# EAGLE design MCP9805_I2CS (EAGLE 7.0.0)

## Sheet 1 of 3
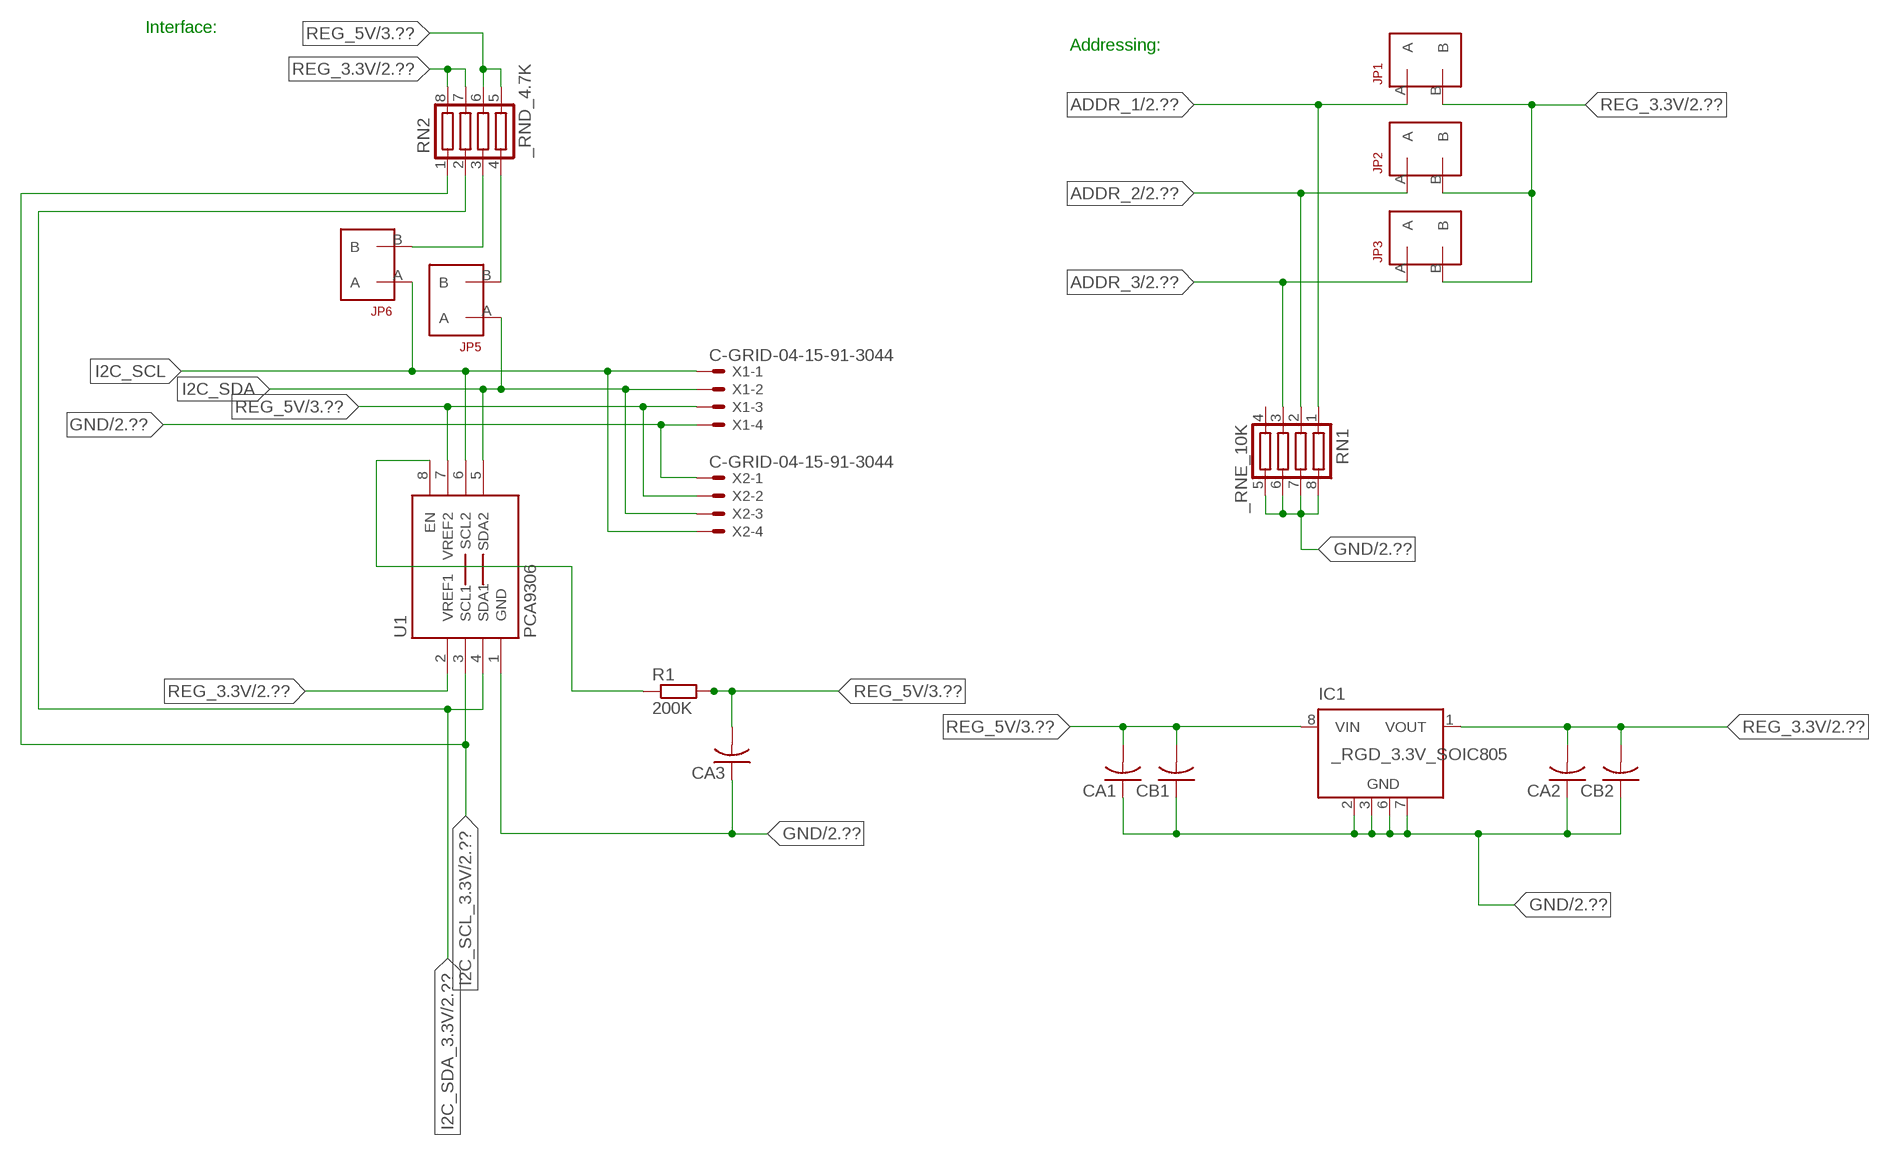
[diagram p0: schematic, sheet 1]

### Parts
CA1  CC1206KRX7R9BB104  [.1UF]
CA2  CC1206KRX7R9BB104  [.1UF]
CA3  CC1206KRX7R9BB104  [.1UF]
CB1  TMK316F106ZL-TC1206K  [TMK316F106ZL-T]
CB2  TMK316F106ZL-TC1206K  [TMK316F106ZL-T]
IC1  _RGD_3.3V_SOIC805  [_RGC_3.3V_SOIC8]
JP1  JUMPER_1X2_2MM  [JUMPER_1X2_2MM]
JP2  JUMPER_1X2_2MM  [JUMPER_1X2_2MM]
JP3  JUMPER_1X2_2MM  [JUMPER_1X2_2MM]
JP5  JUMPER_1X2_2MM  [JUMPER_1X2_2MM]
JP6  JUMPER_1X2_2MM  [JUMPER_1X2_2MM]
R1  200K  RESISTOR_SMT-0603  [R603]
RN1  _RNE_10K  [RNE]
RN2  _RND_4.7K  [RND]
U1  PCA9306  PCA9306_NCD  [PSOP-8]
X1  C-GRID-04-15-91-3044  [15-91-04]
X2  C-GRID-04-15-91-3044  [15-91-04]

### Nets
ADDR_1: JP1.A RN1.1 ; also sheet 2
ADDR_2: JP2.A RN1.2 ; also sheet 2
ADDR_3: JP3.A RN1.3 ; also sheet 2
GND: CA1.1 CA2.1 CA3.1 CB1.1 CB2.1 IC1.2(GND) IC1.3(GND) IC1.6(GND) IC1.7(GND) RN1.5 RN1.6 RN1.7 RN1.8 U1.1(GND) X1.4 X2.1 ; also sheet 2,3
I2C_SCL: JP6.A U1.6(SCL2) X1.1 X2.4
I2C_SCL_3.3V: RN2.1 U1.3(SCL1) ; also sheet 2
I2C_SDA: JP5.A U1.5(SDA2) X1.2 X2.3
I2C_SDA_3.3V: RN2.2 U1.4(SDA1) ; also sheet 2
N$1: JP6.B RN2.3
N$2: JP5.B RN2.4
N$3: R1.1 U1.8(EN)
REG_3.3V: CA2.2 CB2.2 IC1.1(VOUT) JP1.B JP2.B JP3.B RN2.7 RN2.8 U1.2(VREF1) ; also sheet 2
REG_5V: CA1.2 CA3.2 CB1.2 IC1.8(VIN) R1.2 RN2.5 RN2.6 U1.7(VREF2) X1.3 X2.2 ; also sheet 3
Unconnected: IC1.4(NC) IC1.5(NC) RN1.4

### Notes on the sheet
- Interface:
- Addressing:

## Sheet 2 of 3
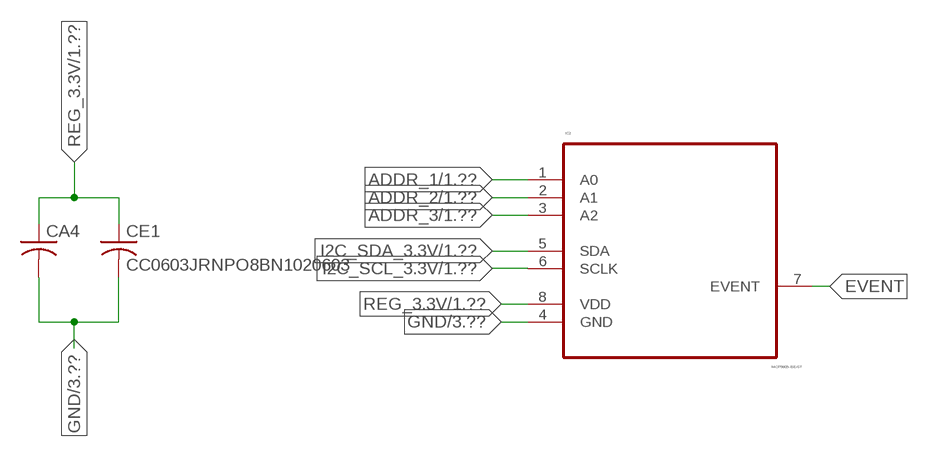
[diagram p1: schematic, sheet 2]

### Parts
CA4  CC1206KRX7R9BB104  [.1UF]
CE1  CC0603JRNPO8BN1020603  [CC0603JRNPO8BN102]
IC2  MCP9805-BE/ST  [SOP65P640X110-8N]

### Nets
ADDR_1: IC2.1(A0) ; also sheet 1
ADDR_2: IC2.2(A1) ; also sheet 1
ADDR_3: IC2.3(A2) ; also sheet 1
EVENT: IC2.7(EVENT)
GND: CA4.2 CE1.2 IC2.4(GND) ; also sheet 1,3
I2C_SCL_3.3V: IC2.6(SCLK) ; also sheet 1
I2C_SDA_3.3V: IC2.5(SDA) ; also sheet 1
REG_3.3V: CA4.1 CE1.1 IC2.8(VDD) ; also sheet 1

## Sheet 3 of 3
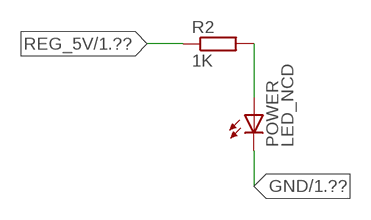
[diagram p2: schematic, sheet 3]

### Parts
POWER  LED_NCD  [CHIPLED_0603]
R2  1K  RESISTOR_SMT-0402  [R402]

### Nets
GND: POWER.C ; also sheet 1,2
N$4: POWER.A R2.2
REG_5V: R2.1 ; also sheet 1

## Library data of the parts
CA1-CA3 = NCD_ULTIMATE_LIBRARY:CC1206KRX7R9BB104: Capacitor CA .1uF 50V SMT C1206K CC1206KRX7R9BB104
CA4 = NCD_ULTIMATE_LIBRARY (2):CC1206KRX7R9BB104: Capacitor CA .1uF 50V SMT C1206K CC1206KRX7R9BB104
CB1 CB2 = NCD_ULTIMATE_LIBRARY:TMK316F106ZL-T: Capacitor CB 10uF SMT 1206 TMK316F106ZL-T
CE1 = NCD_ULTIMATE_LIBRARY (2):CC0603JRNPO8BN102: Capacitor CE 1uF SMT CC0603JRNPO8BN102 0603
IC1 = NCD_ULTIMATE_LIBRARY:_RGD_3.3V_SOIC8: Regulator Linear 3.3V Chip Positive VOLTAGE REGULATOR Digikey 497-1199-2-ND/L78L33ACD13TR
IC2 = NCD_ULTIMATE_KAMNA:MCP9805-BE/ST: SENSOR, TEMP JEDEC +/-1C ACC; MPN: MCP9805-BE/ST; OC_FARNELL: 1439489; OC_NEWARK: -; PACKAGE: SENSOR, TEMP; SUPPLIER: Microchip
JP1-JP3 JP5 JP6 = NCD_ULTIMATE_CONNECTORS:JUMPER_1X2_2MM
POWER = NCD_ULTIMATE_LIBRARY:LED_NCD: LED Digikey 754-1132-2-ND/APT2012SRCPRV
R1 R2 = NCD_ULTIMATE_LIBRARY:RESISTOR_SMT: NCD Resistor
RN1 = NCD_ULTIMATE_LIBRARY:_RNE_10K: Resistor Array RNE SMT 10K x 4 Single Resistor Source: http://www.ctscorp.com/components/Datasheets/CTSChipArrayDs.pdf Digikey 742C083103JPTR-ND/742C083103JP; OC_FARNELL: unknown; OC_NEWARK: unknown
RN2 = NCD_ULTIMATE_LIBRARY:_RND_4.7K: Resistor Array RND SMT 4.7K x 4 Single Resistor Source: http://www.ctscorp.com/components/Datasheets/CTSChipArrayDs.pdf Digikey 742C083472JPTR-ND/742C083472JP; OC_FARNELL: unknown; OC_NEWARK: unknown
U1 = NCD_ULTIMATE_LIBRARY:PCA9306_NCD: NCD Bidirectional I2C level shifter. NOT compatible with all available part number pinout schemes- DOUBLE CHECK!!!; PROD_ID: IC-10023
X1 X2 = NCD_ULTIMATE_CONNECTORS:C-GRID-04: CONNECTOR 4-Pos I2C wire to board 2.54 mm (0.100") pitch header Digikey WM1342-ND/0015912045; OC_FARNELL: unknown; OC_NEWARK: unknown

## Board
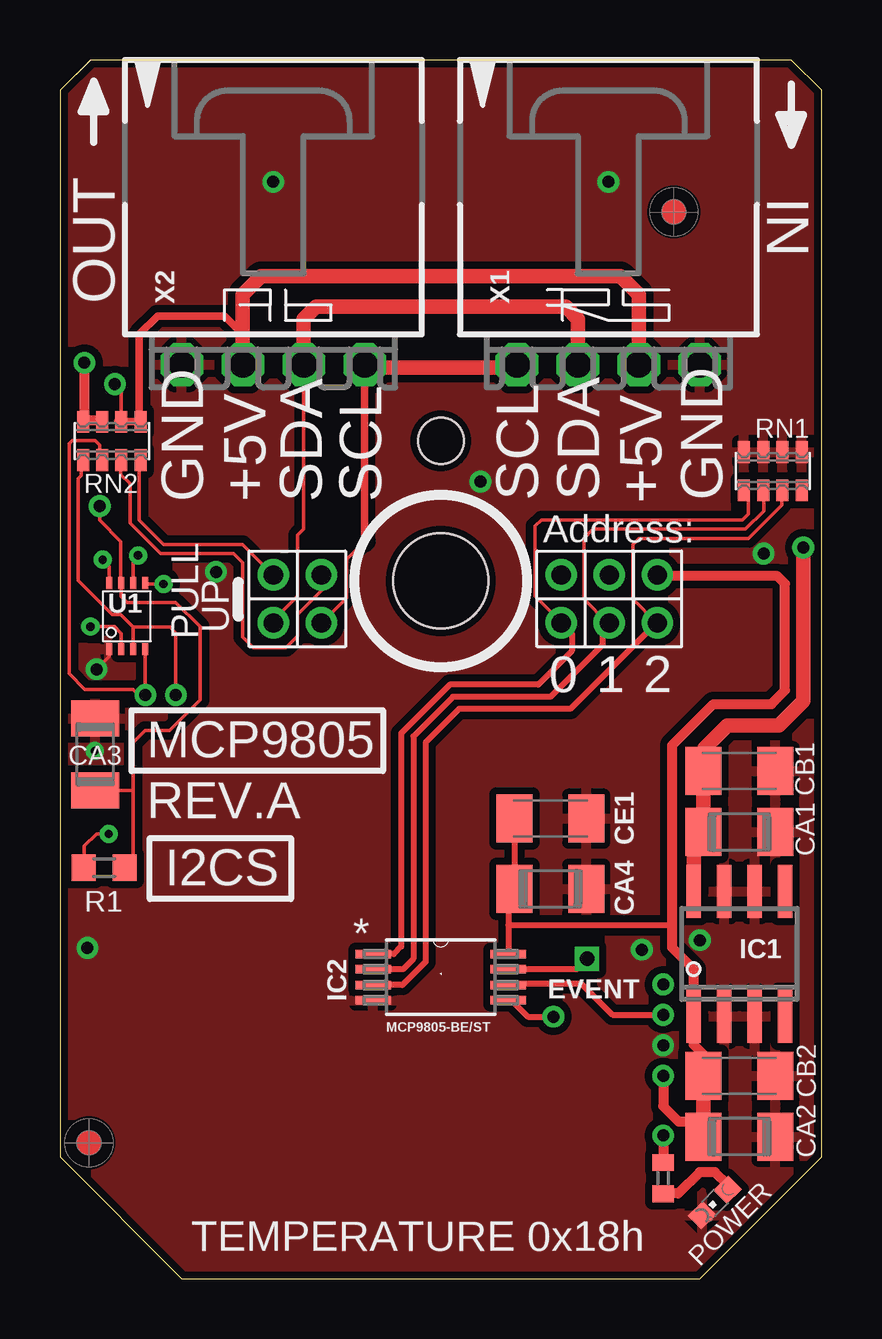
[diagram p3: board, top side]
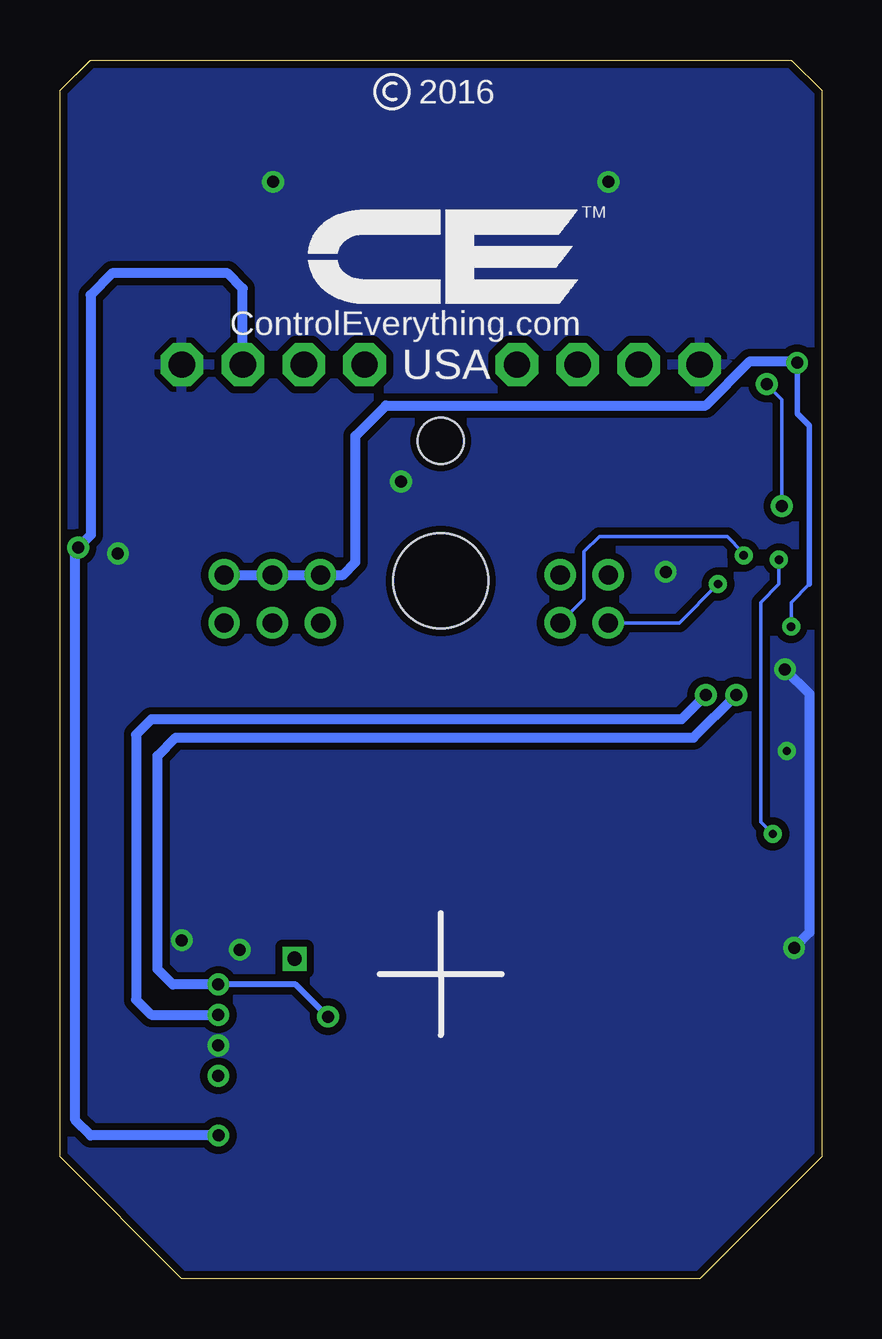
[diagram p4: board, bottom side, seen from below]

Size 31.75 x 50.8 mm. Coordinates in mm from the lower left corner, seen from the top.
Outline: 48 segments
Copper layers (1*16): Top 0.035mm / dielectric 1.5mm / Bottom 0.035mm
Design rules "default": minimum track width 5mil, minimum drill 24mil, track to track 5mil, track to pad 5mil, pad to pad 5mil, via to via 5mil, smd to smd 5mil, copper to edge 10mil, drill to drill 8mil, minimum pad ring 10mil, minimum via ring 8mil, stop-mask expansion 2mil, vias tented up to drill 0mil, thermal gap 10mil
Holes 3.96 mm at 15.88,29.08
Holes 1.91 mm at 15.88,34.93

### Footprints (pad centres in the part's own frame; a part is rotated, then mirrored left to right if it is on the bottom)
.1UF = smd 1.5 x 2: 1 -1.5,0; 2 1.5,0
TMK316F106ZL-T = smd 1.5 x 2: 1 -1.5,0; 2 1.5,0
CC0603JRNPO8BN102 = smd 1.5 x 2: 1 -1.5,0; 2 1.5,0
_RGC_3.3V_SOIC8 = smd 0.6 x 2.2: 1 -1.905,-2.6; 2 -0.635,-2.6; 3 0.635,-2.6; 4 1.905,-2.6; 5 1.905,2.6; 6 0.635,2.6; 7 -0.635,2.6; 8 -1.905,2.6
SOP65P640X110-8N = smd 1.473 x 0.356: 1 -2.819,0.965; 2 -2.819,0.33; 3 -2.819,-0.33; 4 -2.819,-0.965; 5 2.819,-0.965; 6 2.819,-0.33; 7 2.819,0.33; 8 2.819,0.965
JUMPER_1X2_2MM = drill 0.8: A 0,2; B 0,0
CHIPLED_0603 = smd 0.8 x 0.876: A 0,-0.75; C 0,0.75
R603 = smd 1 x 1.1: 1 -0.85,0; 2 0.85,0
R402 = smd 0.7 x 0.9: 1 -0.65,0; 2 0.65,0
RNE = smd 0.5 x 0.9: 1 -1.2,-0.8; 2 -0.4,-0.8; 3 0.4,-0.8; 4 1.2,-0.8; 5 1.2,0.8; 6 0.4,0.8; 7 -0.4,0.8; 8 -1.2,0.8
RND = smd 0.5 x 0.9: 1 -1.2,-0.8; 2 -0.4,-0.8; 3 0.4,-0.8; 4 1.2,-0.8; 5 1.2,0.8; 6 0.4,0.8; 7 -0.4,0.8; 8 -1.2,0.8
PSOP-8 = smd 0.25 x 0.5: 1 -0.73,-1.37; 2 -0.23,-1.37; 3 0.27,-1.37; 4 0.77,-1.37; 5 0.77,1.38; 6 0.27,1.38; 7 -0.23,1.38; 8 -0.73,1.38
15-91-04 = drill 1.1 pad 1.778 octagon: 1 -3.81,-7.62; 2 -1.27,-7.62; 3 1.27,-7.62; 4 3.81,-7.62

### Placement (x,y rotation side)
CA1  28.32,18.62 180 top
CA2  28.32,5.92 180 top
CA3  1.46,21.86 270 top
CA4  20.45,16.26 0 top
CB1  28.32,21.16 180 top
CB2  28.32,8.46 180 top
CE1  20.45,19.18 0 top
IC1  28.32,13.54 0 top
IC2  15.88,12.57 0 top
JP1  20.89,29.34 180 top
JP2  22.9,29.34 180 top
JP3  24.91,29.34 180 top
JP5  8.89,29.34 180 top
JP6  10.9,29.34 180 top
POWER  27.3,3.18 135 top
R1  1.84,17.13 0 top
R2  25.15,4.19 270 top
RN1  29.72,33.66 0 top
RN2  2.16,34.93 0 top
U1  2.79,27.61 0 top
U$5  [VISION_REF10]  1.21,5.66 90 top
U$28  [VISION_REF10]  25.59,44.46 90 top
X1  22.86,45.72 0 top
X2  8.89,45.72 0 top

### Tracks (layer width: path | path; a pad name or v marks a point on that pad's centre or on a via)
ADDR_1
  Top 0.152: JP1.A 20.89,27.37 19.81,28.45 19.81,31.37 20.07,31.62 28.45,31.62 28.7,31.88 28.7,32.78 RN1.1
  Top 0.254: IC2.1 13.92,13.54 14.22,13.84 14.22,22.73 16.26,24.77 19.94,24.77 21.34,26.16 21.34,26.9 JP1.A
ADDR_2
  Top 0.152: JP2.A 22.83,27.34 21.84,28.32 21.84,30.86 22.23,31.24 28.57,31.24 29.34,32 29.34,32.59 RN1.2
  Top 0.254: IC2.2 14.3,12.9 14.73,13.34 14.73,22.61 16.38,24.26 20.45,24.26 22.61,26.42 22.61,27.04 JP2.A
ADDR_3
  Top 0.152: JP3.A 24.86,27.34 23.88,28.32 23.88,30.61 24.13,30.86 28.7,30.86 30.1,32.26 30.1,32.83 RN1.3
  Top 0.254: 24.86,27.34 21.27,23.75 16.64,23.75 15.24,22.35 15.24,13.21 14.28,12.24 IC2.3
EVENT  (via drill 0.6)
  Top 0.254: v21.97,13.34 21.54,12.9 IC2.7
GND  (via drill 0.35, 0.5)
  Top 0.152: CA3.1 1.52,23.42 1.52,23.62 | v1.52,25.4 2.06,25.94 U1.1
  Bottom 0.406: v1.52,25.4 0.51,24.38 0.51,14.43 v1.15,13.79
  other vias: 8.89,45.72 22.86,45.72 25.15,9.73 17.53,33.22 26.67,14.11 6.5,29.46 24.26,13.72 1.45,22 29.34,30.23
  pour Bottom (isolate 0.305): -0.64,5.08 -0.64,49.53 1.27,51.44 30.48,51.44 32.38,49.53 32.38,5.08 26.67,-0.63 5.08,-0.63
  pour Top (isolate 0.305): 4.45,-1.27 -1.27,4.45 -1.27,50.17 0.64,52.07 31.11,52.07 33.02,50.17 33.02,4.45 27.3,-1.27
I2C_SCL  (via drill 0.35)
  Top 0.152: 12.7,30.73 11.94,29.97 11.94,28.38 JP6.A | v3.25,30.15 3.06,29.99 U1.6
  Top 0.305: 12.7,30.73 X2.4
  Top 0.406: X2.4 12.7,37.97 | 19.05,37.97 X1.1
  Top 0.61: 12.7,37.97 19.05,37.97
  Bottom 0.152: JP6.A 9.91,28.33 9.91,30.3 9.27,30.94 3.94,30.94 3.3,30.3 v3.25,30.15
I2C_SCL_3.3V  (via drill 0.5)
  Top 0.152: RN2.1 0.89,34.07 0.89,33.48 0.77,33.35 0.77,29.1 2.17,27.69 2.54,27.69 3.06,27.17 | 3.06,27.17 U1.3 | v4.83,24.33 v4.83,24.34 4.83,26.92 4.58,27.17 3.06,27.17
  Top 0.254: 18.75,12.32 18.77,12.32 | 18.77,12.32 21.72,12.32 23.04,11 v25.15,11 | IC2.6 18.77,12.32
  Bottom 0.406: v4.83,24.33 5.84,23.32 27.94,23.32 28.58,22.68 28.58,11.63 27.94,11 v25.15,11
I2C_SDA  (via drill 0.35)
  Top 0.152: JP5.A 8.89,27.44 9.91,28.45 9.91,30.99 10.16,31.24 10.16,34.92 X2.3 | U1.5 3.6,28.96 v4.32,28.96
  Top 0.61: X2.3 10.16,40.01 10.67,40.51 21.09,40.51 21.59,40.01 X1.2
  Bottom 0.152: v4.32,28.96 5.94,27.34 JP5.A
I2C_SDA_3.3V  (via drill 0.5)
  Top 0.152: RN2.2 1.65,34.14 1.65,34.75 1.46,34.94 0.51,34.94 0.38,34.81 0.38,26.37 0.38,26.36 0.38,25.22 1.04,24.56 3.05,24.56 3.28,24.33 v3.56,24.33 v3.56,24.34 U1.4
  Top 0.254: v20.57,10.92 19.51,10.92 18.82,11.61 IC2.5
  Bottom 0.254: v20.57,10.92 21.92,12.27 v25.15,12.27
  Bottom 0.406: v25.15,12.27 27.05,12.27 27.69,12.9 27.69,21.79 26.93,22.56 5.34,22.56 v3.56,24.33
N$1
  Top 0.152: JP6.B 10.92,29.31 10.92,28.7 9.91,27.69 9.91,26.8 9.42,26.31 8.06,26.31 7.62,26.75 7.62,29.84 7.24,30.23 4.19,30.23 2.92,31.5 2.92,33.15 2.54,33.53 2.54,34.1 RN2.3
  Top 0.305: 2.54,34.02 RN2.3
N$2
  Top 0.152: JP5.B 7.62,30.61 4.32,30.61 3.3,31.62 3.3,34.07 RN2.4
  Top 0.305: 3.37,33.88 RN2.4
N$3  (via drill 0.35)
  Top 0.152: R1.1 1.02,17.16 1.02,18.03 1.52,18.54 v2.03,18.54 | v1.78,29.97 2.06,29.69 U1.8
  Bottom 0.152: v2.03,18.54 2.54,19.05 2.54,28.19 1.78,28.96 v1.78,29.97
N$4
  Top 0.406: POWER.A 27.84,3.92 27.3,4.45 26.67,4.45 25.78,3.56 25.16,3.56 R2.2
REG_3.3V  (via drill 0.35, 0.5)
  Top 0.152: v1.27,27.18 2.29,27.18 2.56,26.9 U1.2
  Top 0.254: 18.64,13.59 IC2.8 18.69,14.73 | CE1.1 CA4.1 18.69,16 18.69,14.73 | 25.53,14.73 18.69,14.73
  Top 0.406: CB2.2 26.82,9.35 26.42,9.75 26.42,10.36 | v25.15,8.46 25.15,7.19 25.78,6.55 26.82,6.55 | IC1.1 26.42,12.9 25.53,13.79 25.53,14.73 25.53,22.24 27.24,23.95 29.66,23.95 30.23,24.52 30.23,28.97 29.91,29.29 24.96,29.29 JP3.B | 26.52,5.62 CA2.2 | v1.02,38.18 1.02,35.78 | 1.02,35.78 RN2.8 | 1.02,35.78 1.71,35.78 RN2.7
  Top 0.61: CB2.2 26.82,6.55 CA2.2 | 26.42,10.36 IC1.1
  Bottom 0.152: 0.51,28.96 1.27,28.19 v1.27,27.18
  Bottom 0.229: 0.51,28.96 0.51,35.56 1.02,36.07 v1.02,38.18
  Bottom 0.406: v1.02,38.18 1.08,38.24 2.99,38.24 4.83,36.4 18.16,36.4 19.43,35.13 19.43,29.87 19.94,29.34 JP1.B JP2.B JP3.B
REG_5V  (via drill 0.5)
  Top 0.152: RN2.6 2.56,37.01 v2.29,37.29 | R1.2 3.05,17.49 3.05,20.36 | 3.05,20.36 3.05,22.35 3.56,22.86 4.57,22.86 5.84,24.13 5.84,27.18 4.83,28.19 2.79,28.19 2.56,28.43 U1.7 2.54,29.01 2.54,30.73 1.65,31.62 v1.65,32.21 | CA3.2 3.05,20.36
  Top 0.305: 7.62,39.37 7.5,39.37 | 2.42,35.74 RN2.6 RN2.5 3.31,35.8 3.31,39.37 4.07,40.13 6.86,40.13 7.62,39.37 | X2.2 7.62,39.37
  Top 0.406: v25.15,5.97 R2.1
  Top 0.61: X1.3 24.13,41.02 23.37,41.78 8.38,41.78 7.62,41.02 X2.2 | IC1.8 26.42,18.21 CA1.2 CB1.2 26.86,21.2 26.86,22.11 27.82,23.06 29.98,23.06 30.99,24.08 v30.99,30.48
  Bottom 0.152: v1.65,32.21 1.65,36.65 v2.29,37.29
  Bottom 0.406: X1.3 24.13,41.28 24.77,41.91 29.58,41.91 30.48,41.01 30.47,31 v30.99,30.48 31.11,30.36 31.11,6.6 30.48,5.97 v25.15,5.97

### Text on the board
tNames: IN | OUT | GND | +5V | SDA | SCL | SCL | SDA | +5V | GND | Address: | PULL | UP | 0 | 1 | 2 | MCP9805 | REV.A | I2CS | EVENT | TEMPERATURE 0x18h
bNames: 2016 | TM | ControlEverything.com | USA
